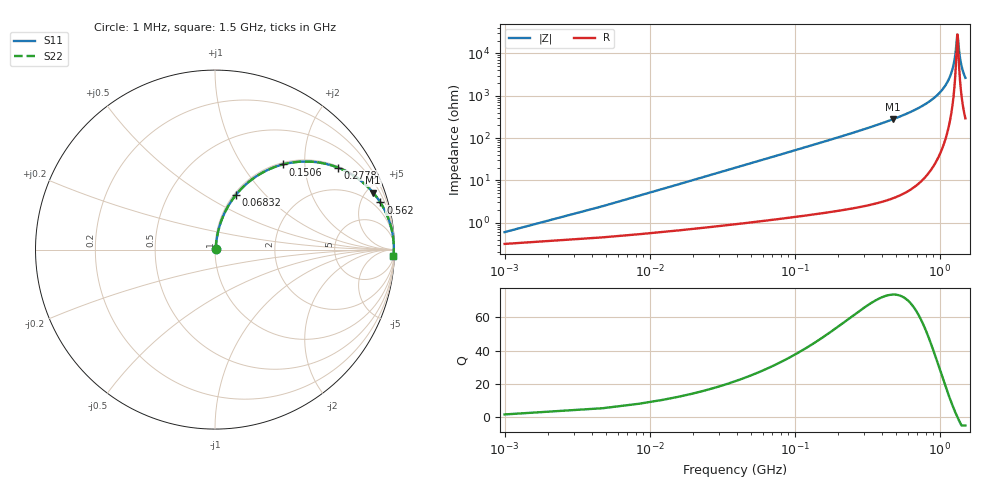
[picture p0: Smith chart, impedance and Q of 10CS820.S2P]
! Coilcraft 1008CS-820 Chip Inductor
! 02 July 2002
# MHZ S MA R 50
!Freq  MagS11  AngS11  MagS21  AngS21  MagS12  AngS12  MagS22  AngS22
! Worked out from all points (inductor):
!   402 points, 1 MHz to 1.5 GHz, reference 50 ohm
!   read as one part in series: L = 81 nH near 8.48 MHz
!   highest Q = 73.6 at 472.2 MHz (marker M1), where L = 92.8 nH
!   self-resonance near 1.321 GHz
!   S11 on the Smith chart (normalised r, x): 1 MHz: 1.01, +0.01; 68.32 MHz: 1.02, +0.70; 150.6 MHz: 1.03, +1.55; 277.8 MHz: 1.05, +2.96; 562 MHz: 1.10, +6.98; 1.5 GHz: 7, -52
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1  0.005966 58.0  0.9968 -0.3  0.9968 -0.3  0.005966 58.0
12.22  0.062 80.9  0.9921 -3.5  0.9921 -3.5  0.062 80.9
19.7  0.09933 80.3  0.9881 -5.7  0.9881 -5.7  0.09933 80.3
38.4  0.1905 76.4  0.9728 -11.0  0.9728 -11.0  0.1905 76.4
68.32  0.326 69.1  0.9346 -19.0  0.9346 -19.0  0.326 69.1
150.6  0.6072 51.4  0.7818 -37.4  0.7818 -37.4  0.6072 51.4
251.58  0.7928 36.6  0.5967 -52.4  0.5967 -52.4  0.7928 36.6
277.76  0.8225 33.8  0.5561 -55.3  0.5561 -55.3  0.8225 33.8
472.24  0.9359 19.9  0.3397 -69.4  0.3397 -69.4  0.9359 19.9
502.16  0.9444 18.4  0.3162 -70.8  0.3162 -70.8  0.9444 18.4
562  0.9578 15.9  0.2743 -73.3  0.2743 -73.3  0.9578 15.9
752.74  0.9819 10.0  0.1732 -79.0  0.1732 -79.0  0.9819 10.0
1003.32  0.9937 4.7  0.08253 -83.2  0.08253 -83.2  0.9937 4.7
1160.4  0.9961 2.2  0.03882 -83.1  0.03882 -83.1  0.9961 2.2
1253.9  0.9965 0.9  0.01601 -76.9  0.01601 -76.9  0.9965 0.9
1280.08  0.9965 0.5  0.01013 -69.6  0.01013 -69.6  0.9965 0.5
1321.22  0.9964 0.0  0.003564 -2.6  0.003564 -2.6  0.9964 0.0
1332.44  0.9964 -0.1  0.00429 33.0  0.00429 33.0  0.9964 -0.1
1366.1  0.9963 -0.6  0.01041 68.6  0.01041 68.6  0.9963 -0.6
1396.02  0.9961 -0.9  0.01659 75.9  0.01659 75.9  0.9961 -0.9
1440.9  0.9957 -1.5  0.02583 79.7  0.02583 79.7  0.9957 -1.5
1500  0.9951 -2.1  0.03769 81.5  0.03769 81.5  0.9951 -2.1
